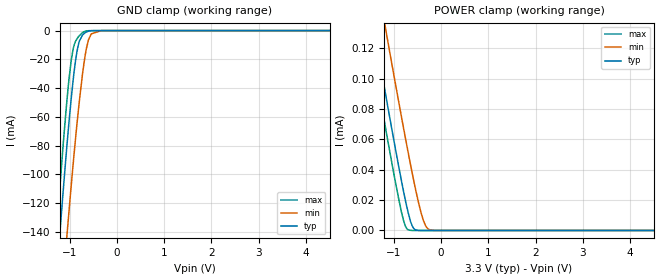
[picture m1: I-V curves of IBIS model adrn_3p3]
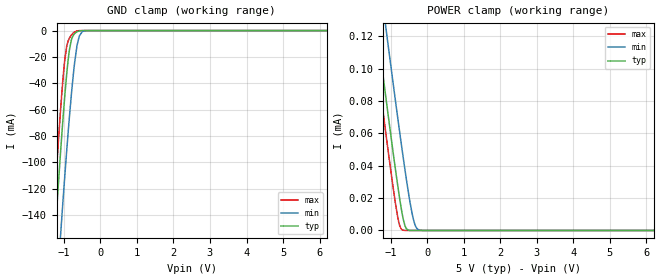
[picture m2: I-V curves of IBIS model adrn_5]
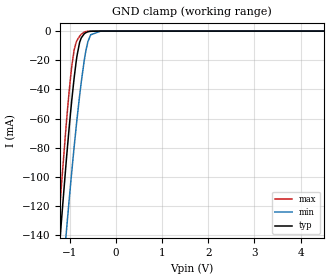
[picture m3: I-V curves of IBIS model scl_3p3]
|Texas Instruments Incorporated
| Low Power, High Accuracy Humidity Sensor with Integrated Digital Temperature
| Sensor
| Marketing part#   Digital Voltage Range   Package-type   #pins
| HDC1000YPAR   2.7V-5.5V   DSBGA   8
| HDC1000YPAT   2.7V-5.5V   DSBGA   8
| HDC1010YPAR   2.7V-5.5V   DSBGA   8
| HDC1010YPAT   2.7V-5.5V   DSBGA   8
| HDC1008YPAR   2.7V-5.5V   DSBGA   8
| HDC1008YPAT   2.7V-5.5V   DSBGA   8
| HDC1080DMBR   2.7V-5.5V   VSON   6
| HDC1080DMBT   2.7V-5.5V   VSON   6
[IBIS Ver]   4.1
[File name]   hdc100x.ibs
[File Rev]   1.1
[Date]   08/18/2016
[Source]
| Texas Instruments Incorporated.
| Analog-eLab Design Center, HPA
| 12500 TI Blvd
| Dallas, TX -75243
[Notes]   Revision History:
| Rev 1.1: 08/18/2016
| - Add component name HDC1010 and HVD1080 to reflect new product offering
| Rev 1.0: 11/05/2014
| - Initial version of the model
| - Model generated from simulations in SPECTRE
| - Model matched to SPICE simulation
| - C_comp although listed in numerical order of value are
|   obtained from varying PVT conditions. For PVT conditions for
|   each specific value refer the buffer description under
|   respective [Model]. IBIS model user is responsible for using
|   appropriate C_comp to simulate for Signal Integrity.
[Disclaimer]
| This model is designed as an aid for customers of Texas Instruments.
| TI and its licensors and suppliers make no warranties, either expressed
| or implied, with respect to this  model, including the warranties of
| merchantability or fitness for a particular purpose. The model is
| provided solely on an "as is" basis. The entire risk as to its quality
| and performance is with the customer.
[Copyright]
(C) Copyright 2016 Texas Instruments Incorporated.All rights reserved.
|   HDC1000YPA
[Component]   HDC1000YPA
[Manufacturer]   TI
[Package]   |8 DSBGA  -  YPA package
|   typ   min   max
R_pkg   0.00500   0.00500   0.00500
L_pkg   0.20000nH   0.20000nH   0.20000nH
C_pkg   0.60000pF   0.60000pF   0.60000pF
[Pin]  signal_name   model_name   R_pin   L_pin   C_pin
A1   SCL   SCL   0.00500   0.20000nH  0.60000pF
B1   VDD   POWER   0.00500   0.20000nH  0.60000pF
C1   ADR0   ADRN   0.00500   0.20000nH  0.60000pF
D1   ADR1   ADRN   0.00500   0.20000nH  0.60000pF
A2   SDA   SDA   0.00500   0.20000nH  0.60000pF
B2   GND   GND   0.00500   0.20000nH  0.60000pF
C2   DNC   NC   0.00500   0.20000nH  0.60000pF
D2   DRDYn   DRDYn   0.00500   0.20000nH  0.60000pF
|   HDC1010YPA
[Component]   HDC1010YPA
[Manufacturer]   TI
[Package]   |8 DSBGA  -  YPA package
|   typ   min   max
R_pkg   0.00500   0.00500   0.00500
L_pkg   0.20000nH   0.20000nH   0.20000nH
C_pkg   0.60000pF   0.60000pF   0.60000pF
[Pin]  signal_name   model_name   R_pin   L_pin   C_pin
A1   SCL   SCL   0.00500   0.20000nH  0.60000pF
B1   VDD   POWER   0.00500   0.20000nH  0.60000pF
C1   ADR0   ADRN   0.00500   0.20000nH  0.60000pF
D1   ADR1   ADRN   0.00500   0.20000nH  0.60000pF
A2   SDA   SDA   0.00500   0.20000nH  0.60000pF
B2   GND   GND   0.00500   0.20000nH  0.60000pF
C2   DNC   NC   0.00500   0.20000nH  0.60000pF
D2   DRDYn   DRDYn   0.00500   0.20000nH  0.60000pF
|   HDC1008YPA
[Component]   HDC1008YPA
[Manufacturer]   TI
[Package]   |8 DSBGA  -  YPA package
|   typ   min   max
R_pkg   0.00500   0.00500   0.00500
L_pkg   0.20000nH   0.20000nH   0.20000nH
C_pkg   0.60000pF   0.60000pF   0.60000pF
[Pin]  signal_name   model_name   R_pin   L_pin   C_pin
A1   SCL   SCL   0.00500   0.20000nH  0.60000pF
B1   VDD   POWER   0.00500   0.20000nH  0.60000pF
C1   ADR0   ADRN   0.00500   0.20000nH  0.60000pF
D1   ADR1   ADRN   0.00500   0.20000nH  0.60000pF
A2   SDA   SDA   0.00500   0.20000nH  0.60000pF
B2   GND   GND   0.00500   0.20000nH  0.60000pF
C2   DNC   NC   0.00500   0.20000nH  0.60000pF
D2   DRDYn   DRDYn   0.00500   0.20000nH  0.60000pF
|   HDC1080DMB
[Component]   HDC1080DMB
[Manufacturer]   TI
[Package]   |6 PWSON  -  DMB package
|   typ   min   max
R_pkg   0.00500   0.00500   0.00500
L_pkg   0.20000nH   0.20000nH   0.20000nH
C_pkg   0.60000pF   0.60000pF   0.60000pF
[Pin]  signal_name   model_name   R_pin   L_pin   C_pin
1   SDA   SDA   0.00500   0.20000nH  0.60000pF
2   GND   GND   0.00500   0.20000nH  0.60000pF
3   NC   NC   0.00500   0.20000nH  0.60000pF
4   NC   NC   0.00500   0.20000nH  0.60000pF
5   VDD   POWER   0.00500   0.20000nH  0.60000pF
6   SCL   SCL   0.00500   0.20000nH  0.60000pF
|   Model Selectors
[Model Selector] SCL
scl_3p3   3.3V  digital Input
scl_5   5.0V  digital Input
[Model Selector] ADRN
adrn_3p3   3.3V digital Input
adrn_5   5.0V digital Input
[Model Selector] DRDYn
drdyn_3p3   3.3V digital Open_drain
drdyn_5   5.0V digital Open_drain
[Model Selector] SDA
sda_3p3   3.3V digital I/O_open_drain
sda_5   5.0V digital I/O_open_drain
| Models and submodels in the file (8): adrn_3p3 (Input), adrn_5 (Input), scl_3p3 (Input), scl_5 (Input), drdyn_3p3 (Open_drain), drdyn_5 (Open_drain), sda_3p3 (I/O_open_drain), sda_5 (I/O_open_drain)
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|   adrn_3p3 Model
[Model]   adrn_3p3
Model_type   Input
Vinl = 0.99
Vinh = 2.31
|   typ   min   max
|   (nom PVT)   (fast PVT)   (slow PVT)
C_comp   4.581e-13   4.355e-13   5.484e-13
[Model spec]
|subparameter
Vinl   0.99   0.90   1.08
Vinh   2.31   2.10   2.52
| Where nom  PVT is Nominal Process, 3.3V, 27C
|   Fast PVT is Strong Process,  3.6V, -40C
|   Slow PVT is Weak Process,   3V, 150C
[Voltage Range]   3.3   3   3.6
|Junction Temperature
[Temperature Range]   27   150   -40
[Power Clamp Reference]   3.3   3   3.6
[GND Clamp Reference]   0   0   0
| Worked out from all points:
|   GND clamp passes 1 mA (typ) near -0.65 V on its own axis
[GND Clamp]
|   Voltage   I(typ)   I(min)   I(max)
-3.3V     -1.112A    -1.143A    -1.099A
-1.281V   -173.7mA   -235.5mA   -142.1mA
-1.239V   -155.4mA   -217.7mA   -123.4mA
-1.144V   -114.9mA   -177.9mA   -82.48mA
-1.064V   -83.01mA   -145.9mA   -51.4mA
-1.036V   -72.25mA   -134.8mA   -41.43mA
-963mV    -46.38mA   -106.8mA   -20.05mA
-844.8mV  -14.62mA   -65.22mA   -5.723mA
-686.4mV  -1.804mA   -20.52mA   -702.9uA
-543mV    -121uA     -2.294mA   -14.52uA
-330mV    -331.4nA   -27.51uA   0A
6.6V      0A         0A         0A
[POWER Clamp]
|   Voltage   I(typ)   I(min)   I(max)
-3.3V     475.5uA    516.8uA    454.3uA
-1.575V   161uA      203.9uA    138.8uA
-1.383V   126.6uA    169.7uA    104.3uA
-1.139V   83.5uA     126.6uA    61.19uA
-838.2mV  32.74uA    74.91uA    12.23uA
-762.3mV  20.99uA    62.23uA    3.517uA
-699mV    12.11uA    51.86uA    524.5nA
-574.2mV  1.166uA    32.24uA    0A
-425.7mV  0A         11.94uA    0A
-330mV    0A         3.329uA    0A
-225mV    0A         335.7nA    0A
6.6V      0A         0A         0A
|   adrn_5 Model
[Model]   adrn_5
Model_type   Input
Vinl = 1.5
Vinh = 3.5
|   typ   min   max
|   (nom PVT)   (fast PVT)   (slow PVT)
C_comp   4.581e-13   4.355e-13   5.484e-13
[Model spec]
|subparameter
Vinl   1.5   1.35   1.65
Vinh   3.5   3.15   3.85
| Where nom  PVT is Nominal Process, 5V, 27C
|   Fast PVT is Strong Process,  5.5V, -40C
|   Slow PVT is Weak Process,   4.5V, 150C
[Voltage Range]   5   4.5   5.5
|Junction Temperature
[Temperature Range]   27   150   -40
[Power Clamp Reference]   5   4.5   5.5
[GND Clamp Reference]   0   0   0
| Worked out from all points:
|   GND clamp passes 1 mA (typ) near -0.65 V on its own axis
[GND Clamp]
|   Voltage   I(typ)   I(min)   I(max)
-5V       -1.902A    -1.913A    -1.903A
-1.353V   -205.1mA   -265.9mA   -174.1mA
-1.265V   -166mA     -228.1mA   -134.1mA
-1.18V    -129.4mA   -192.4mA   -96.97mA
-1.075V   -86.48mA   -149.5mA   -54.62mA
-974mV    -49.48mA   -110.4mA   -22.24mA
-882.5mV  -22.46mA   -77.4mA    -7.94mA
-800mV    -7.793mA   -50.51mA   -3.662mA
-639.5mV  -852.8uA   -11.36mA   -228uA
-500mV    -40.44uA   -958.3uA   -3.231uA
-360.5mV  -812nA     -51.81uA   -16.15nA
10V       0A         0A         0A
[POWER Clamp]
|   Voltage   I(typ)   I(min)   I(max)
-5V       788.3uA    828.4uA    767.6uA
-1.505V   148.2uA    191.3uA    126uA
-1.254V   103.7uA    146.9uA    81.32uA
-1.172V   89.16uA    132.4uA    66.84uA
-1.067V   70.98uA    114.1uA    48.79uA
-814.5mV  28.81uA    70.8uA     9.127uA
-666.5mV  8.05uA     46.49uA    222nA
-565mV    895.4nA    30.72uA    0A
-396.5mV  0A         8.644uA    0A
-302mV    0A         1.906uA    0A
-194mV    0A         161nA      0A
10V       0A         0A         0A
|   scl_3p3 Model
[Model]   scl_3p3
Model_type   Input
Vinl = 0.99
Vinh = 2.31
|   typ   min   max
|   (nom PVT)   (fast PVT)   (slow PVT)
C_comp   4.581e-13   4.355e-13   5.484e-13
[Model spec]
|subparameter
Vinl   0.99   0.90   1.08
Vinh   2.31   2.10   2.52
| Where nom  PVT is Nominal Process, 3.3V, 27C
|   Fast PVT is Strong Process,  3.6V, -40C
|   Slow PVT is Weak Process,   3V, 150C
[Voltage Range]   3.3   3   3.6
|Junction Temperature
[Temperature Range]   27   150   -40
[Power Clamp Reference]   3.3   3   3.6
[GND Clamp Reference]   0   0   0
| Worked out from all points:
|   GND clamp passes 1 mA (typ) near -0.64 V on its own axis
[GND Clamp]
|   Voltage   I(typ)   I(min)   I(max)
-3.3V     -1.109A    -1.088A    -1.129A
-1.302V   -181.8mA   -225.7mA   -160.1mA
-1.188V   -134mA     -181mA     -109.9mA
-1.066V   -85.94mA   -135.2mA   -60.51mA
-980.1mV  -55.59mA   -104.8mA   -31.43mA
-906mV    -32.85mA   -80.22mA   -13.47mA
-785.4mV  -7.811mA   -44.37mA   -3.524mA
-686.4mV  -1.93mA    -20.42mA   -731.1uA
-606mV    -488.1uA   -7.307mA   -98.06uA
-546mV    -131.1uA   -2.528mA   -16.03uA
-330mV    -332.2nA   -27.49uA   0A
6.6V      0A         0A         0A
[POWER Clamp]
|   Voltage   I(typ)   I(min)   I(max)
-3.3V     0A         0A         0A
0V        0A         0A         0A
6.6V      0A         0A         0A
